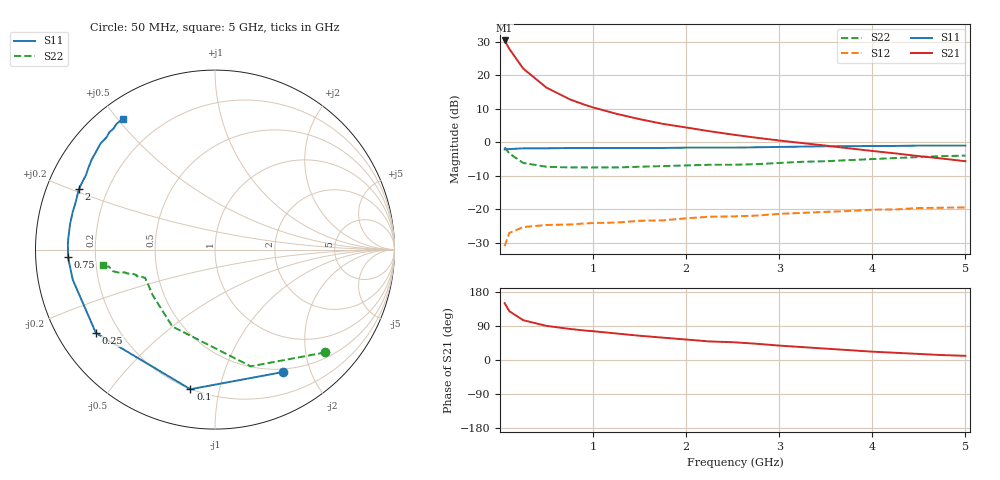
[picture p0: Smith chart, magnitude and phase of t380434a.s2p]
!AT-38043
!S-PARAMETERS at Vce=3.6V Ic=50mA. LAST UPDATED 01-06-98
# ghz s ma r 50
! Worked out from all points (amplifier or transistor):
!   23 points, 50 MHz to 5 GHz, reference 50 ohm
!   highest |S21| = 30.4 dB at 50 MHz (marker M1)
!   |S21| within 3 dB of that: start of sweep to 112.7 MHz
!   unconditionally stable (mu >= 1): 1.596 GHz to end of sweep
!   at 500 MHz: K = 0.40, MSG = 20.5 dB, |S12| = -24.7 dB
!   at 2.25 GHz: K = 1.16, MAG = 10.4 dB, |S12| = -22.3 dB
!   at 5 GHz: K = 1.30, MAG = 3.6 dB, |S12| = -19.5 dB
!   S11 on the Smith chart (normalised r, x): 50 MHz: 0.46, -1.60; 100 MHz: 0.20, -0.82; 250 MHz: 0.12, -0.31; 750 MHz: 0.10, -0.03; 2 GHz: 0.10, +0.21; 5 GHz: 0.07, +0.52
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0.05  0.78 -61.0  33.11 150.0  0.028 54.0  0.84 -43.0
0.1  0.79 -100.0  24.83 129.0  0.044 42.0  0.68 -73.0
0.25  0.81 -145.0  12.59 105.0  0.054 24.0  0.49 -119.0
0.5  0.81 -168.0  6.53 90.0  0.058 20.0  0.43 -144.0
0.75  0.82 -177.0  4.37 82.0  0.059 19.0  0.42 -153.0
0.9  0.82 178.0  3.67 78.0  0.061 22.0  0.42 -155.0
1  0.82 176.0  3.31 76.0  0.062 23.0  0.42 -156.0
1.25  0.82 170.0  2.66 70.0  0.063 24.0  0.42 -158.0
1.5  0.82 165.0  2.21 64.0  0.067 28.0  0.43 -159.0
1.75  0.82 161.0  1.88 59.0  0.068 30.0  0.44 -160.0
2  0.83 156.0  1.66 54.0  0.073 32.0  0.45 -161.0
2.25  0.83 152.0  1.46 49.0  0.077 34.0  0.46 -161.0
2.5  0.83 150.0  1.3 47.0  0.078 39.0  0.46 -162.0
2.75  0.84 147.0  1.17 43.0  0.08 40.0  0.47 -163.0
3  0.85 144.0  1.06 38.0  0.085 43.0  0.49 -164.0
3.5  0.87 137.0  0.89 30.0  0.091 45.0  0.52 -166.0
3.75  0.87 134.0  0.81 26.0  0.094 45.0  0.54 -166.0
4  0.88 132.0  0.74 22.0  0.098 46.0  0.56 -167.0
4.25  0.88 130.0  0.68 19.0  0.099 46.0  0.58 -168.0
4.5  0.89 128.0  0.62 16.0  0.104 46.0  0.6 -171.0
4.75  0.89 126.0  0.57 13.0  0.105 46.0  0.62 -171.0
5  0.89 125.0  0.52 11.0  0.106 46.0  0.63 -172.0
